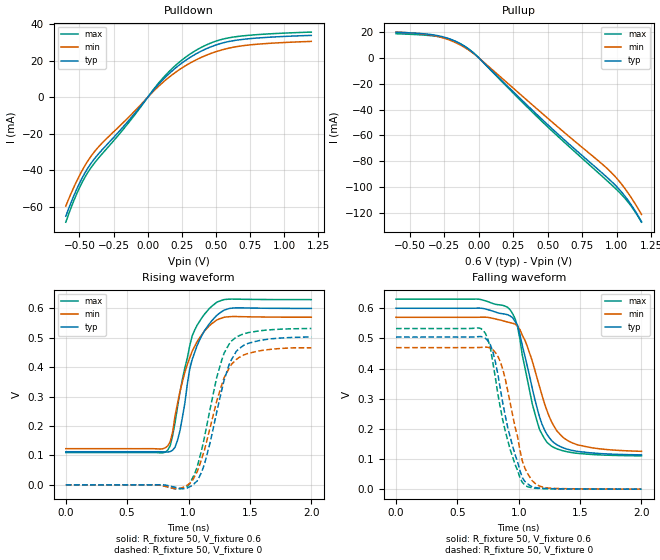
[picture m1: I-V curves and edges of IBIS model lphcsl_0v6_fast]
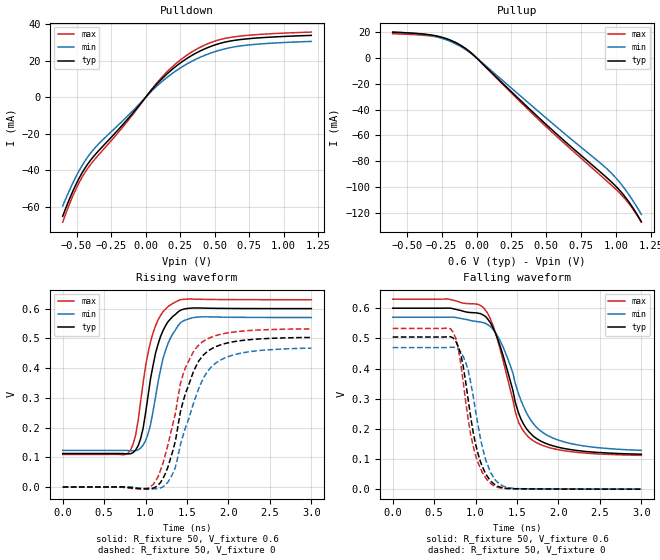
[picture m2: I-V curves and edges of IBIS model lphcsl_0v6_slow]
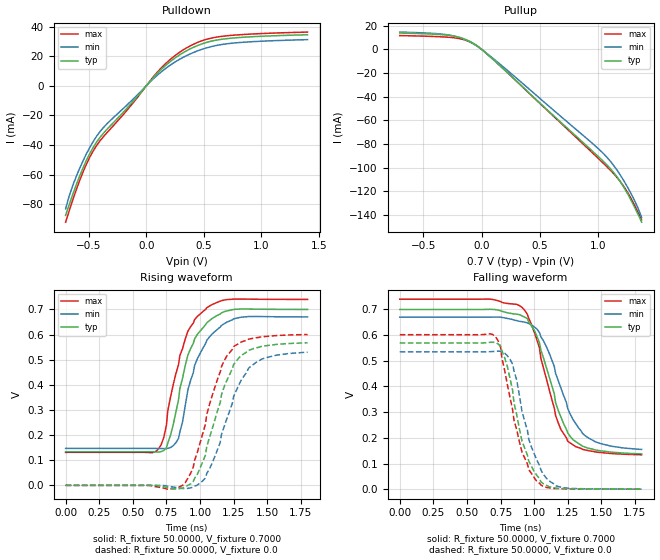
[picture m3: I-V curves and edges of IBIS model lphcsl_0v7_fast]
| Integrated Devices Technolgy, Inc
[IBIS Ver]   4.2
[File name]   9dbv0831.ibs
[File Rev]   1.5
|Rev history   1.5   Update Ref models with different slew-rate setting 08-17-2015
|Rev history   1.4   09-27-2013 update LP_HCSP model
|Rev history   1.3   08-14 update IN data
|Rev history   1.2   08-14 update ^CKPWRGD_PD# data
|Rev history   1.1   08-13 update CLKIN data
|Rev history   1.0   original revision
[Date]   27 Aug, 2015
[Disclaimer] Integrated Device Technology, Inc. ("IDT") hereby grants the
   user of this ibis model a non-exclusive, nontransferable
   license to use this ibis model under the following terms. the
   user is granted this license only to use the ibis model and is
   not granted rights to sell, copy (except as needed to run the
   ibis model), rent, lease or sub-license the ibis model in
   whole or in part, or in modified form to anyone. the user may
   modify the ibis model to suit its specific applications, but
   rights to derivative works and such modifications shall belong
   to idt. this ibis model is provided on an as is" basis and idt
   makes absolutely no warranty with respect to the information
   contained herein. idt disclaims and customer waives all
   warranties, express and implied, including warranties of
   merchantability and fitness for a particular purpose. the
   entire risk as to quality and performance is with the user
   accordingly, in no event shall idt be liable for any direct or
   indirect damages, whether in contract or tort, including any
   lost profits or other incidental, consequential, exemplary, or
   punitive damages arising out of the use or application of the
   ibis model. further, idt reserves the right to make changes
   without notice to any product herein to improve reliability,
   function, or design. idt does not convey any license under
   patent rights or any other intellectual property rights,
   including those of third parties. idt is not obligated to
   provide maintenance or support for the licensed ibis model.
[Copyright]   Copyright 2012, Integrated Devices Technolgy, Inc. all rights
   reserved
[Component]   9DBV0831
[Manufacturer] Integrated Device Technology, Inc.
[Package]
R_pkg   72.4655m   58.886m   86.045m
L_pkg   1.47175nH   1.11650nH   1.77850nH
C_pkg   0.07747pF   0.07444pF   0.08050pF
[Pin] signal_name  model_name
1 vSADR_tri   IN
2 ^vHIBW_BYPM_LOBW#   IN
3 FB_DNC   LP_HCSL
4 FB_DNC#   LP_HCSL
5 VDDR1.8   POWER
6 CLK_IN   CLKIN
7 CLK_IN#   CLKIN
8 GNDR   GND
9 GNDDIG   GND
10 SCLK_3.3   SCIN
11 SDATA_3.3   SCIN
12 VDDDIG1.8   POWER
13 VDDIO   POWER
14 vOE0#   IN
15 DIF0   LP_HCSL
16 DIF0#   LP_HCSL
17 vOE1#   IN
18 DIF1   LP_HCSL
19 DIF1#   LP_HCSL
20 VDD1.8   POWER
21 VDDIO   POWER
22 GND   GND
23 DIF2   LP_HCSL
24 DIF2#   LP_HCSL
25 vOE2#   IN
26 DIF3   LP_HCSL
27 DIF3#   LP_HCSL
28 vOE3#   IN
29 GNDA   GND
30 VDDA1.8   POWER
31 VDDIO   POWER
32 DIF4   LP_HCSL
33 DIF4#   LP_HCSL
34 vOE4#   IN
35 DIF5   LP_HCSL
36 DIF5#   LP_HCSL
37 vOE5#   IN
38 VDD1.8   POWER
39 VDDIO   POWER
40 GND   GND
41 DIF6   LP_HCSL
42 DIF6#   LP_HCSL
43 vOE6#   IN
44 DIF7   LP_HCSL
45 DIF7#   LP_HCSL
46 vOE7#   IN
47 VDDIO   POWER
48 ^CKPWRGD_PD#   PD
49 EPAD   GND
[Diff Pin]  inv_pin  vdiff tdelay_typ tdelay_min  tdelay_max
3   4   NA   0   0   0
15   16   NA   0   0   0
18   19   NA   0   0   0
23   24   NA   0   0   0
26   27   NA   0   0   0
32   33   NA   0   0   0
35   36   NA   0   0   0
41   42   NA   0   0   0
44   45   NA   0   0   0
[Model Selector] LP_HCSL
lphcsl_0v6_fast amplitude 0.6V, slew rate fast
lphcsl_0v6_slow amplitude 0.6V, slew rate slow
lphcsl_0v7_fast amplitude 0.7V, slew rate fast
lphcsl_0v7_slow amplitude 0.7V, slew rate slow
lphcsl_0v8_fast amplitude 0.8V, slew rate fast
lphcsl_0v8_slow amplitude 0.8V, slew rate slow
lphcsl_0v9_fast amplitude 0.9V, slew rate fast
lphcsl_0v9_slow amplitude 0.9V, slew rate slow
| Models and submodels in the file (12): lphcsl_0v6_fast (Output), lphcsl_0v6_slow (Output), lphcsl_0v7_fast (Output), lphcsl_0v7_slow (Output), lphcsl_0v8_fast (Output), lphcsl_0v8_slow (Output), lphcsl_0v9_fast (Output), lphcsl_0v9_slow (Output), SCIN (Input), IN (Input), CLKIN (Input), PD (Input)
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[Model]   lphcsl_0v6_fast
Model_type Output
Polarity Non-Inverting
Enable Active-High
Vmeas = 0.4000V
Cref = 2.0000pF
Rref = 0
Vref = 0.4000V
C_comp 1.1000pF 1.0000pF 1.2000pF
[Temperature Range] 25 75 0
[Voltage Range] 0.6000V 0.5700V 0.6300V
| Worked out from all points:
|   slope of the pulldown table from 0 to 0.09 V, typ, clamps not added: 11.3 ohm
|   slope of the pullup table from 0 to 0.09 V, typ, clamps not added: 9.48 ohm
|   rising waveform, R_fixture 50, V_fixture 0.6: 20-80 % time 160ps typ, 180ps min, 159ps max; typ from 0.113 V to 0.6 V
|   rising waveform, R_fixture 50, V_fixture 0: 20-80 % time 176ps typ, 190ps min, 173ps max; typ from 0 V to 0.503 V
|   falling waveform, R_fixture 50, V_fixture 0.6: 20-80 % time 180ps typ, 217ps min, 161ps max; typ from 0.6 V to 0.114 V
|   falling waveform, R_fixture 50, V_fixture 0: 20-80 % time 163ps typ, 145ps min, 164ps max; typ from 0.504 V to 0 V
[Pulldown]
|Voltage I(typ) I(min) I(max)
-600mV    -65.21mA   -59.64mA   -68.48mA
-540mV    -53.77mA   -49.11mA   -56.45mA
-500mV    -47.15mA   -42.93mA   -49.62mA
-440mV    -38.96mA   -35.03mA   -41.34mA
-380mV    -32.74mA   -28.88mA   -35.09mA
-140mV    -12.81mA   -10.93mA   -13.94mA
100mV     8.769mA    7.433mA    9.577mA
260mV     19.34mA    16.56mA    21mA
420mV     26.34mA    22.82mA    28.41mA
580mV     30.41mA    26.74mA    32.45mA
800mV     32.55mA    29.15mA    34.41mA
1.2V      34.02mA    30.72mA    35.83mA
[Pullup]
|Voltage I(typ) I(min) I(max)
-600mV    19.81mA    19.9mA     18.63mA
-380mV    18.39mA    18.13mA    17.44mA
-260mV    16.25mA    15.47mA    15.78mA
-160mV    12.32mA    11.36mA    12.3mA
-60mV     5.642mA    5.048mA    5.78mA
0V        720.8pA    1.104nA    645pA
480mV     -49.7mA    -44.85mA   -51.38mA
940mV     -93.39mA   -86.48mA   -95.95mA
1V        -99.57mA   -93.12mA   -101.9mA
1.06V     -107mA     -101.1mA   -108.6mA
1.12V     -116mA     -110.5mA   -116.9mA
1.18V     -126.7mA   -121.1mA   -127.1mA
[Ramp]
| variable typ min max
dV/dt_r 0.3017/0.1766n 0.2797/0.1900n 0.3191/0.1728n
dV/dt_f 0.2917/0.1873n 0.2666/0.2169n 0.3116/0.1771n
R_load = 50
[Rising Waveform]
R_fixture= 50
V_fixture= 0.6
V_fixture_min= 0.57
V_fixture_max= 0.63
|time V(typ) V(min) V(max)
0s        112.6mV    123mV      109.7mV
810ps     111.8mV    125.8mV    111.1mV
850ps     113.2mV    146mV      132.5mV
910ps     151.4mV    276.4mV    264.1mV
970ps     277.8mV    382.9mV    397.8mV
1.01ns    394.9mV    432.9mV    473.6mV
1.03ns    426.8mV    454.8mV    507.4mV
1.17ns    548.2mV    541.3mV    600.3mV
1.33ns    599.8mV    571.9mV    631.7mV
2ns       600.1mV    570.3mV    630.1mV
[Rising Waveform]
R_fixture= 50
V_fixture= 0
V_fixture_min= 0
V_fixture_max= 0
|time V(typ) V(min) V(max)
0s        0V         0V         0V
990ps     -10.88mV   -1.163mV   -4.753mV
1.07ns    13.16mV    43.5mV     60.52mV
1.13ns    70.91mV    118.7mV    162.5mV
1.23ns    248.4mV    285.1mV    366.2mV
1.29ns    356mV      364.6mV    448.2mV
1.35ns    426.1mV    410.1mV    489.3mV
1.39ns    454.8mV    426.7mV    503.1mV
1.49ns    482mV      447.8mV    518.2mV
2ns       502.9mV    466.2mV    531.9mV
[Falling Waveform]
R_fixture= 50
V_fixture= 0.6
V_fixture_min= 0.57
V_fixture_max= 0.63
|time V(typ) V(min) V(max)
0s        600mV      570mV      630mV
670ps     600.4mV    570.1mV    630.3mV
910ps     578.4mV    554.2mV    603mV
990ps     544mV      540.9mV    539.4mV
1.05ns    441.8mV    494.3mV    403.9mV
1.15ns    268.4mV    367.7mV    224.1mV
1.23ns    181.9mV    260.5mV    155.5mV
1.31ns    147.6mV    193.6mV    133.8mV
1.43ns    129.2mV    154.7mV    121.6mV
2ns       113.8mV    125.6mV    110.6mV
[Falling Waveform]
R_fixture= 50
V_fixture= 0
V_fixture_min= 0
V_fixture_max= 0
|time V(typ) V(min) V(max)
0s        504.4mV    469.5mV    532.8mV
710ps     504.7mV    470.8mV    527mV
750ps     491.6mV    470.5mV    495.3mV
790ps     455.1mV    462mV      418.3mV
850ps     333.2mV    423.2mV    270.3mV
950ps     142.8mV    246.4mV    106.9mV
1.03ns    38.06mV    92.3mV     21.97mV
1.07ns    19.06mV    53.05mV    8.341mV
1.23ns    2.108mV    4.368mV    1.591mV
2ns       93.89uV    172.9uV    66.57uV
[Model]   lphcsl_0v6_slow
Model_type Output
Polarity Non-Inverting
Enable Active-High
Vmeas = 0.4000V
Cref = 2.0000pF
Rref = 0
Vref = 0.4000V
C_comp 1.1000pF 1.0000pF 1.2000pF
[Temperature Range] 25 75 0
[Voltage Range] 0.6000V 0.5700V 0.6300V
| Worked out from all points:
|   slope of the pulldown table from 0 to 0.09 V, typ, clamps not added: 11.3 ohm
|   slope of the pullup table from 0 to 0.09 V, typ, clamps not added: 9.48 ohm
|   rising waveform, R_fixture 50, V_fixture 0.6: 20-80 % time 199ps typ, 206ps min, 195ps max; typ from 0.113 V to 0.6 V
|   rising waveform, R_fixture 50, V_fixture 0: 20-80 % time 296ps typ, 331ps min, 287ps max; typ from 0 V to 0.503 V
|   falling waveform, R_fixture 50, V_fixture 0.6: 20-80 % time 326ps typ, 384ps min, 300ps max; typ from 0.6 V to 0.116 V
|   falling waveform, R_fixture 50, V_fixture 0: 20-80 % time 195ps typ, 202ps min, 192ps max; typ from 0.504 V to 0 V
[Pulldown]
|Voltage I(typ) I(min) I(max)
-600mV    -65.21mA   -59.64mA   -68.48mA
-540mV    -53.77mA   -49.11mA   -56.45mA
-500mV    -47.15mA   -42.93mA   -49.62mA
-440mV    -38.96mA   -35.03mA   -41.34mA
-380mV    -32.74mA   -28.88mA   -35.09mA
-140mV    -12.81mA   -10.93mA   -13.94mA
100mV     8.769mA    7.433mA    9.577mA
260mV     19.34mA    16.56mA    21mA
420mV     26.34mA    22.82mA    28.41mA
580mV     30.41mA    26.74mA    32.45mA
800mV     32.55mA    29.15mA    34.41mA
1.2V      34.02mA    30.72mA    35.83mA
[Pullup]
|Voltage I(typ) I(min) I(max)
-600mV    19.81mA    19.9mA     18.63mA
-380mV    18.39mA    18.13mA    17.44mA
-260mV    16.25mA    15.47mA    15.78mA
-160mV    12.32mA    11.36mA    12.3mA
-60mV     5.642mA    5.048mA    5.78mA
0V        720.8pA    1.104nA    645pA
480mV     -49.7mA    -44.85mA   -51.38mA
940mV     -93.39mA   -86.48mA   -95.95mA
1V        -99.57mA   -93.12mA   -101.9mA
1.06V     -107mA     -101.1mA   -108.6mA
1.12V     -116mA     -110.5mA   -116.9mA
1.18V     -126.7mA   -121.1mA   -127.1mA
[Ramp]
| variable typ min max
dV/dt_r 0.3017/0.3160n 0.2800/0.3389n 0.3190/0.3071n
dV/dt_f 0.2905/0.3464n 0.2648/0.4039n 0.3107/0.3200n
R_load = 50
[Rising Waveform]
R_fixture= 50
V_fixture= 0.6
V_fixture_min= 0.57
V_fixture_max= 0.63
|time V(typ) V(min) V(max)
0s        112.6mV    123mV      109.7mV
820ps     111.9mV    122.2mV    125.1mV
880ps     124.2mV    122.2mV    174.9mV
940ps     162.2mV    131.1mV    287.5mV
1.06ns    364.7mV    209.7mV    488.6mV
1.18ns    505.9mV    393.6mV    576.4mV
1.3ns     565.3mV    500.7mV    612.6mV
1.42ns    594.6mV    552.1mV    629.8mV
1.58ns    602.2mV    570mV      632mV
3ns       600.1mV    570.1mV    630mV
[Rising Waveform]
R_fixture= 50
V_fixture= 0
V_fixture_min= 0
V_fixture_max= 0
|time V(typ) V(min) V(max)
0s        0V         0V         0V
1.09ns    -3.871mV   -6.154mV   8.187mV
1.21ns    28.55mV    413.1uV    79.77mV
1.33ns    123.2mV    46.45mV    212.5mV
1.42ns    252.6mV    142.5mV    346.7mV
1.48ns    314.1mV    199.3mV    400.5mV
1.7ns     444.6mV    367.1mV    490.7mV
1.85ns    472.4mV    417.7mV    509.5mV
2.06ns    488.6mV    444.1mV    521.2mV
3ns       502.9mV    466.7mV    531.7mV
[Falling Waveform]
R_fixture= 50
V_fixture= 0.6
V_fixture_min= 0.57
V_fixture_max= 0.63
|time V(typ) V(min) V(max)
0s        600mV      570mV      630mV
670ps     600.3mV    570.1mV    630.2mV
1.09ns    577.6mV    552.1mV    603.4mV
1.18ns    551.5mV    539.1mV    562.9mV
1.27ns    495.3mV    505.6mV    491.2mV
1.42ns    357.8mV    408.8mV    328.5mV
1.52ns    251.4mV    314.8mV    220.9mV
1.7ns     174.8mV    216.3mV    159.6mV
2.09ns    133.8mV    155.2mV    126.6mV
3ns       115.9mV    128.7mV    112.2mV
[Falling Waveform]
R_fixture= 50
V_fixture= 0
V_fixture_min= 0
V_fixture_max= 0
|time V(typ) V(min) V(max)
0s        504.4mV    469.5mV    532.8mV
730ps     501.1mV    470.9mV    520.3mV
790ps     473.6mV    463.9mV    468.8mV
820ps     449.2mV    455mV      418.4mV
910ps     298mV      395.1mV    234.1mV
970ps     190.3mV    310.2mV    143.9mV
1.09ns    69.97mV    130.9mV    51.15mV
1.21ns    20.11mV    42.35mV    12.74mV
1.48ns    1.492mV    2.259mV    1.252mV
3ns       109.5uV    165.3uV    86.38uV
[Model]   lphcsl_0v7_fast
Model_type Output
Polarity   Non-Inverting
Enable   Active-High
Vmeas =  0.4000V
Cref =   2.0000pF
Rref =   0.0
Vref =   0.4000V
C_comp   1.1000pF   1.0000pF   1.2000pF
[Temperature Range]   25.0000   75.0000   0.0
[Voltage Range]   0.7000V   0.6700V   0.7400V
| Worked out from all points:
|   slope of the pulldown table from 0 to 0.105 V, typ, clamps not added: 11.5 ohm
|   slope of the pullup table from 0 to 0.105 V, typ, clamps not added: 11.5 ohm
|   rising waveform, R_fixture 50.0000, V_fixture 0.7000: 20-80 % time 161ps typ, 172ps min, 163ps max; typ from 0.134 V to 0.7 V
|   rising waveform, R_fixture 50.0000, V_fixture 0.0: 20-80 % time 196ps typ, 209ps min, 193ps max; typ from 0 V to 0.567 V
|   falling waveform, R_fixture 50.0000, V_fixture 0.7000: 20-80 % time 198ps typ, 226ps min, 186ps max; typ from 0.7 V to 0.138 V
|   falling waveform, R_fixture 50.0000, V_fixture 0.0: 20-80 % time 148ps typ, 157ps min, 158ps max; typ from 0.57 V to 0 V
[Pulldown]
|Voltage   I(typ)   I(min)   I(max)
-700mV    -87.46mA   -83.06mA   -92.05mA
-640mV    -73.75mA   -67.7mA    -77.54mA
-580mV    -61.27mA   -56.03mA   -64.32mA
-490mV    -45.66mA   -41.53mA   -48.1mA
-430mV    -37.82mA   -33.91mA   -40.19mA
-340mV    -29.28mA   -25.55mA   -31.55mA
50mV      4.609mA    3.896mA    5.041mA
230mV     17.65mA    15.08mA    19.19mA
410mV     26mA       22.5mA     28.05mA
590mV     30.57mA    26.92mA    32.6mA
860mV     32.86mA    29.49mA    34.71mA
1.4V      34.46mA    31.17mA    36.26mA
[Pullup]
|Voltage   I(typ)   I(min)   I(max)
-700mV    13.69mA    14.51mA    11.54mA
-370mV    12.52mA    13.09mA    10.63mA
-220mV    10.82mA    10.77mA    9.497mA
-100mV    6.649mA    6.27mA     6.197mA
-10mV     821.9uA    747.4uA    796.9uA
290mV     -26.07mA   -23.65mA   -26.13mA
1.04V     -94.6mA    -87.89mA   -96.18mA
1.13V     -104.2mA   -98.2mA    -105.1mA
1.22V     -117.1mA   -111.6mA   -116.4mA
1.31V     -133.6mA   -128mA     -131.9mA
1.34V     -139.7mA   -134.5mA   -137.9mA
1.37V     -146.2mA   -142.3mA   -144.3mA
[Ramp]
| variable   typ   min   max
dV/dt_r  0.3404/0.1944n   0.3179/0.2062n   0.3601/0.1919n
dV/dt_f  0.3375/0.1959n   0.3091/0.2218n   0.3636/0.1855n
R_load = 50.0000
[Rising Waveform]
R_fixture= 50.0000
V_fixture= 0.7000
V_fixture_min= 0.6700
V_fixture_max= 0.7400
|time   V(typ)   V(min)   V(max)
0s        133.6mV    147.2mV    131.3mV
640ps     133.6mV    147.2mV    130.1mV
730ps     139.3mV    146.3mV    190.1mV
780ps     199mV      150.6mV    350.3mV
840ps     340.8mV    187.2mV    480.7mV
910ps     519.1mV    380.8mV    613.9mV
980ps     601mV      504mV      672.2mV
1.09ns    664.1mV    602.6mV    719.7mV
1.25ns    700.2mV    662.9mV    741.4mV
1.8ns     700.2mV    670.4mV    740.1mV
[Rising Waveform]
R_fixture= 50.0000
V_fixture= 0.0
V_fixture_min= 0.0
V_fixture_max= 0.0
|time   V(typ)   V(min)   V(max)
0s        0V         0V         0V
870ps     -10.37mV   -12.56mV   -102.8uV
950ps     16.06mV    -6.886mV   73.86mV
1.04ns    120.1mV    29.51mV    243.5mV
1.07ns    189.3mV    65.39mV    320.9mV
1.16ns    361.1mV    203.1mV    473.5mV
1.25ns    481.3mV    354.1mV    552.7mV
1.36ns    537mV      466mV      581.7mV
1.42ns    547.6mV    490.7mV    587.7mV
1.8ns     567.3mV    529.9mV    600.2mV
[Falling Waveform]
R_fixture= 50.0000
V_fixture= 0.7000
V_fixture_min= 0.6700
V_fixture_max= 0.7400
|time   V(typ)   V(min)   V(max)
0s        700mV      670mV      740mV
670ps     700.5mV    670.1mV    740.3mV
910ps     675.2mV    652.5mV    708.4mV
950ps     664.7mV    647.9mV    680.9mV
1.04ns    569.5mV    609.9mV    549.2mV
1.16ns    336.4mV    450.4mV    286.8mV
1.25ns    219mV      314.3mV    186.5mV
1.36ns    167.7mV    217.5mV    155.1mV
1.45ns    153.3mV    185.8mV    145.6mV
1.8ns     137.5mV    154.9mV    134mV
[Falling Waveform]
R_fixture= 50.0000
V_fixture= 0.0
V_fixture_min= 0.0
V_fixture_max= 0.0
|time   V(typ)   V(min)   V(max)
0s        569.8mV    535.1mV    601.7mV
710ps     571.3mV    536.8mV    595.1mV
750ps     557.2mV    537.2mV    554.1mV
840ps     385.3mV    487mV      309.2mV
850ps     337.3mV    461.6mV    269.4mV
910ps     187mV      302.9mV    144.2mV
960ps     109.8mV    195mV      76.57mV
1.07ns    20.83mV    57.2mV     9.671mV
1.22ns    2.418mV    5.906mV    1.792mV
1.8ns     214uV      374.6uV    155.2uV
